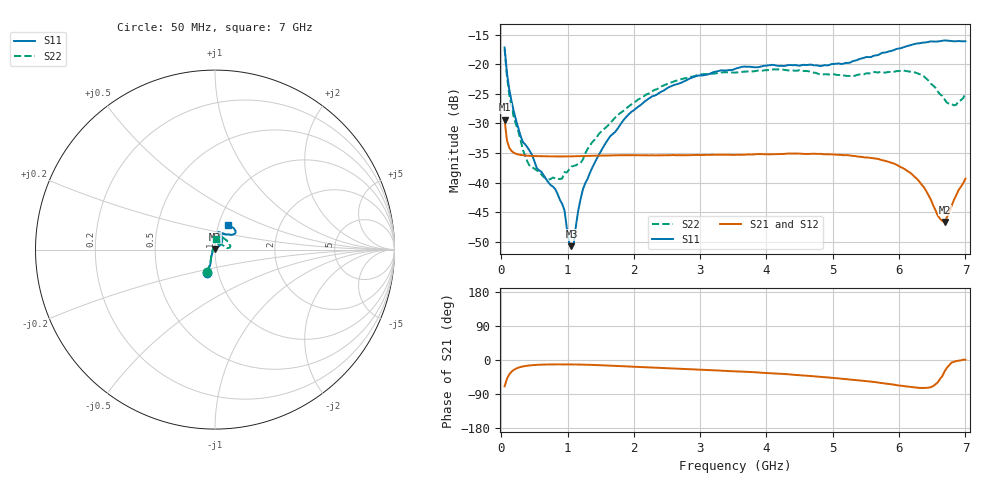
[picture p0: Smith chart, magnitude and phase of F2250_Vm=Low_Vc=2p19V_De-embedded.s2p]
! Integrated Device Technology
! Corporate Headquarters
! 6024 Silver Creek Valley Road
! San Jose, CA 95138  USA
! Phone:  1-408-284-8200
! Toll Free:  1-800-223-1366
! Webpage:  http://www.idt.com/
! Timing and RF Division
! 515 Groton Road, Suite 102
! Westford, MA 01886-6024
! Device:  F2250
! Description: Voltage Variable RF Attenuator
! Frequency:  50.0 -  6000.00 MHz
! Package:  3x3 mm Thin QFN Plastic Package: 16 pin
! Ports:  2 RF, 3 DC
!  Pin  1  = GND
!  Pin  2  = NC
!  Pin  3  = RF1  = Port 1
!  Pin  4  = NC
!  Pin  5  = GND
!  Pin  6  = GND
!  Pin  7  = GND
!  Pin  8  = GND
!  Pin  9  = NC
!  Pin 10  = RF2  = Port 2
!  Pin 11  = NC
!  Pin 12  = GND
!  Pin 13  = GND
!  Pin 14  = VCNTRL
!  Pin 15  = VDD
!  Pin 16  = VMODE
! Vcntrl:  2.190 Volts
! Vmode:  +0.000 Volts
! Vdd:  +3.30  Volts
! Current:  1.179 mA
! Data:  The device was measured on a the F2250 evaluation board which has
!  individual transmission lines to the RF pins.  Data was collected
!  using a calibrated network analyzer.  The evaluation board was
!  de-embedded using a TRL calibration technique.
!  The reference plane is the edge of the package pin.
! Misc:  SN 10
!  Action Tracker AT0258
! Date Measured:  2014-11-26
! Date:  2015-10-15  MJV
! Note:
!  Integrated Device Technology supplies this data as a sample of measured
!  data at the package pin for this product.  Your particular data for this
!  product may vary.
!  Data was taken at 25 degrees C.
!  Integrated Device Technology reserves the right to change this data at anytime.
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# GHz S dB R 50
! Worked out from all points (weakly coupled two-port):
!   201 points, 50 MHz to 7 GHz, reference 50 ohm
!   highest |S21| = -29.38 dB at 50 MHz (marker M1); lowest = -46.7 dB at 6.687 GHz (marker M2)
!   lowest |S11| = -50.7 dB at 1.058 GHz (marker M3), VSWR 1.01, Z = 49.8 + j0.246 ohm
!   |S11| at or under -10 dB: start of sweep to end of sweep
!   |S22| runs from -39.5 to -17.4 dB; largest |S21 - S12| = 6.3e-05
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0.05  -17.18 -108.6  -29.38 -69.4  -29.37 -69.4  -17.42 -110.4
0.08475  -21.44 -107.4  -32.85 -50.0  -32.84 -50.0  -21.95 -108.6
0.189  -27.99 -119.7  -34.96 -26.1  -34.96 -26.1  -28.96 -123.2
0.328  -33.18 -133.7  -35.38 -16.9  -35.38 -16.9  -34.52 -139.8
0.43225  -34.72 -144.7  -35.48 -14.2  -35.48 -14.2  -37.26 -164.6
0.71025  -39.96 -168.4  -35.57 -11.8  -35.57 -11.8  -39.50 152.7
0.91875  -43.61 158.1  -35.58 -11.6  -35.58 -11.6  -39.30 124.7
0.9535  -44.70 170.0  -35.58 -11.6  -35.58 -11.6  -38.23 123.2
1.023  -50.11 144.5  -35.57 -11.6  -35.57 -11.7  -37.79 105.9
1.05775  -50.74 121.9  -35.56 -11.7  -35.56 -11.7  -37.27 100.6
1.0925  -50.37 90.8  -35.55 -11.8  -35.55 -11.8  -37.19 95.5
1.162  -44.61 56.7  -35.54 -11.9  -35.53 -12.0  -36.79 84.4
1.2315  -41.11 44.2  -35.50 -12.2  -35.51 -12.2  -36.10 75.1
1.6485  -32.10 41.9  -35.42 -14.8  -35.42 -14.8  -29.87 59.2
2.37825  -24.87 47.3  -35.38 -20.4  -35.38 -20.5  -24.04 54.1
3.525  -20.80 72.5  -35.31 -29.8  -35.31 -29.8  -21.42 73.4
4.7065  -20.17 72.4  -35.12 -42.8  -35.12 -42.8  -21.42 71.5
5.85325  -17.82 40.5  -36.55 -63.5  -36.54 -63.6  -21.31 21.6
6.27025  -16.51 40.1  -39.37 -72.8  -39.37 -72.8  -21.51 8.3
6.68725  -15.99 48.8  -46.65 -29.7  -46.62 -29.3  -25.97 27.3
6.861  -16.12 55.1  -42.15 -2.8  -42.11 -2.7  -26.85 58.0
7  -16.12 63.3  -39.34 0.7  -39.31 0.6  -24.91 84.1
